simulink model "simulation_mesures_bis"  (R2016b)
settings: Solver=ode15s  StartTime=0.0  StopTime=35*3600  RelTol=1e-3  EnableMultiTasking=on
undefined symbols (not defined in the file or in its folder): C0, C1, Icc, Nbre, Qair, Qpanne, R, R_iso, sigbuilder_block, Time2, V, V0, V1
libraries: powerlib_meascontrol x1, simulink x1

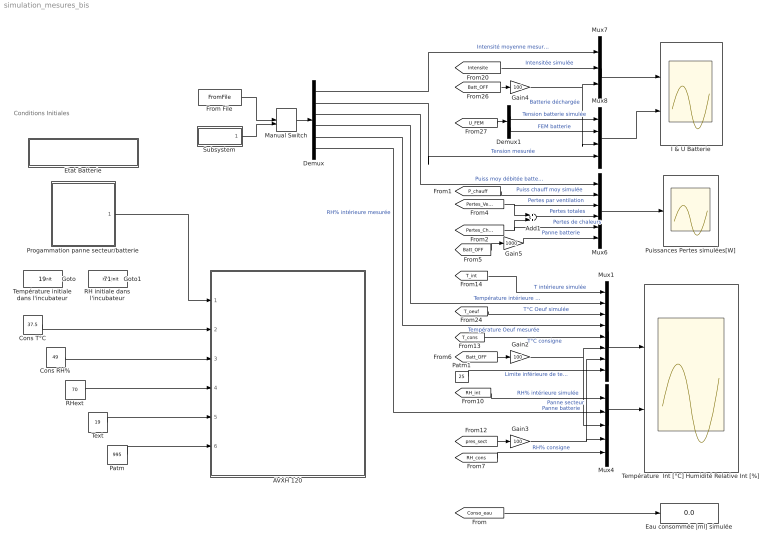
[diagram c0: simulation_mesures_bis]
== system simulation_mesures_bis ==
  note: Conditions Initiales
  AVXH 120 : Subsystem
  Add1 : Sum
  Cons RH% : Constant  Value=49
  Cons T°C : Constant  Value=37.5
  Demux : Demux  Outputs=6
  Demux1 : Demux  Outputs=2
  Eau consommée |ml] simulée : Display
  Etat Batterie : Subsystem  DialogController=hmiCreateDDGDialog  IsWebBlock=on
  From File : FromFile  FileName=mesures1.mat  SampleTime=1
  Gain2 : Gain  Gain=100
  Gain3 : Gain  Gain=100
  Gain4 : Gain  Gain=100
  Gain5 : Gain  Gain=1000
  I & U Batterie : Scope  NumInputPorts=2
  Manual Switch : ManualSwitch
  Mux1 : Mux  Inputs=8
  Mux4 : Mux  Inputs=5
  Mux6 : Mux  Inputs=6
  Mux7 : Mux  Inputs=3
  Mux8 : Mux
  Patm : Constant  Value=995
  Patm1 : Constant  Value=25
  Progammation panne secteur/batterie : Subsystem
  Puissances Pertes simulées[W] : Scope
  RH initiale dans l'incubateur : Constant  Value=71
  RHext : Constant  Value=70
  Subsystem : Subsystem
  Température  Int [°C] Humidité Relative Int [%] : Scope  NumInputPorts=2
  Température initiale dans l'incubateur : Constant  Value=19
  Text : Constant  Value=19
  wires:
  Patm1/1 -> Mux1/8  "Limite inférieure de température"
  Cons T°C/1 -> AVXH 120/2(In2)
  Cons RH%/1 -> AVXH 120/3(In3)
  RHext/1 -> AVXH 120/4(In4)
  Text/1 -> AVXH 120/5(In5)
  Patm/1 -> AVXH 120/6(In6)
  [Conso_eau] -> Eau consommée |ml] simulée/1
  Progammation panne secteur/batterie/1(Out1) -> AVXH 120/1(In1)
  Manual Switch/1 -> Demux/1
  Demux/4 -> Mux1/2  "Température intérieure mesurée"
  Demux/5 -> Mux1/4  "Température Oeuf mesurée"
  Demux/6 -> Mux4/2  "RH% intérieure mesurée"
  [T_int] -> Mux1/1  "T intérieure simulée"
  [Intensite] -> Mux7/2  "Intensitée simulée"
  [RH_int] -> Mux4/1  "RH% intérieure simulée"
  Gain3/1 -> Mux4/4, Mux1/7  "Panne secteur"
  [pres_sect] -> Gain3/1
  [Batt_OFF] -> Gain2/1
  Gain2/1 -> Mux4/3, Mux1/6  "Panne batterie"
  Demux1/1 -> Mux8/1  "Tension batterie simulée"
  [T_cons] -> Mux1/5  "T°C consigne"
  Mux4/1 -> Température  Int [°C] Humidité Relative Int [%]/2
  [P_chauff] -> Mux6/2  "Puiss chauff moy simulée"
  [Pertes_Vent] -> Mux6/3, Add1/1  "Pertes par ventilation"
  Mux6/1 -> Puissances Pertes simulées[W]/1
  [Pertes_Chaleur] -> Mux6/5, Add1/2  "Pertes de chaleurs"
  Add1/1 -> Mux6/4  "Pertes totales"
  [T_oeuf] -> Mux1/3  "T°C Oeuf simulée"
  [RH_cons] -> Mux4/5  "RH% consigne"
  Mux7/1 -> I & U Batterie/1
  Mux8/1 -> I & U Batterie/2
  [U_FEM] -> Demux1/1
  Demux1/2 -> Mux8/2  "FEM batterie"
  [Batt_OFF] -> Gain4/1
  Gain4/1 -> Mux8/3, Mux7/3  "Batterie déchargée"
  [Batt_OFF] -> Gain5/1
  Gain5/1 -> Mux6/6  "Panne batterie"
  Mux1/1 -> Température  Int [°C] Humidité Relative Int [%]/1
  Demux/2 -> Mux8/4  "Tension mesurée"
  Température initiale dans l'incubateur/1 -> [T_init]
  RH initiale dans l'incubateur/1 -> [RH_init]
  Demux/1 -> Mux7/1  "Intensité moyenne mesurée"
  Demux/3 -> Mux6/1  "Puiss moy débitée batterie mesurée"
  From File/1 -> Manual Switch/1
  Subsystem/1(Out1) -> Manual Switch/2

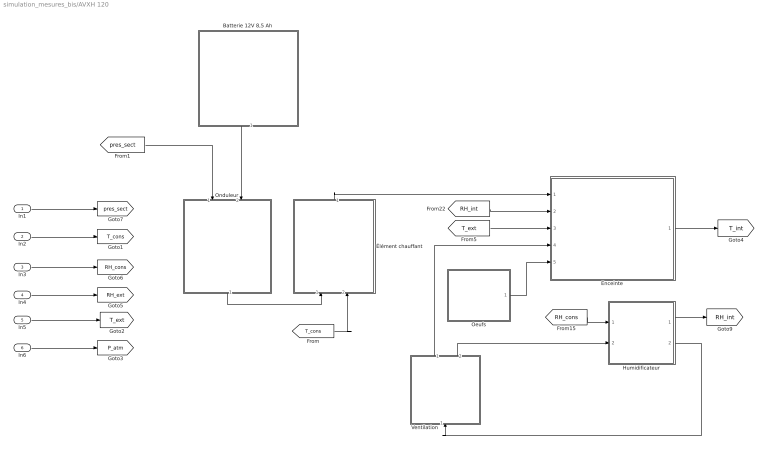
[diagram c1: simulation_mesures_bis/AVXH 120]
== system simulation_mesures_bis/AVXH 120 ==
  In1 : Inport
  In2 : Inport  Port=2
  In3 : Inport  Port=3
  In4 : Inport  Port=4
  In5 : Inport  Port=5
  In6 : Inport  Port=6
  Batterie 12V 8,5 Ah : Subsystem
  Enceinte : Subsystem
  Humidificateur : Subsystem
  Oeufs : Subsystem
  Onduleur : Subsystem
  Ventilation : Subsystem
  Élément chauffant : Subsystem
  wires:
  [RH_int] -> Enceinte/2(In2)
  Enceinte/1(T°C in) -> [T_int]
  In1/1 -> [pres_sect]
  In6/1 -> [P_atm]
  In5/1 -> [T_ext]
  [T_ext] -> Enceinte/3(T°C ext)
  In4/1 -> [RH_ext]
  In3/1 -> [RH_cons]
  Oeufs/1(Out1) -> Enceinte/5(M.Cp_Oeuf)
  [pres_sect] -> Onduleur/1(In1)
  Élément chauffant/1(Out2) -> Enceinte/1(P_chauff)
  Ventilation/1(Out1) -> Enceinte/4(Pertes ventilation)
  [RH_cons] -> Humidificateur/1(In1)
  Ventilation/2(Out2) -> Humidificateur/2(In2)
  Humidificateur/2(Out2) -> Ventilation/1(In1)
  In2/1 -> [T_cons]
  Batterie 12V 8,5 Ah/1(Out3) -> Onduleur/2(In2)
  Onduleur/1(Out1) -> Élément chauffant/1(In1)
  [T_cons] -> Élément chauffant/2(In2)
  Humidificateur/1(Out1) -> [RH_int]

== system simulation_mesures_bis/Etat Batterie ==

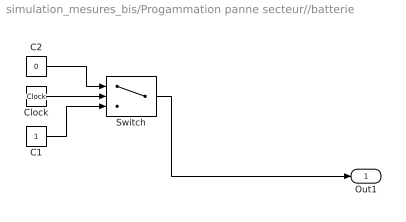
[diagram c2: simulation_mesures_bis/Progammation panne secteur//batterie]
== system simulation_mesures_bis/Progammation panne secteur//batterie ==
  C1 : Constant
  C2 : Constant  Value=0
  Clock : Clock
  Switch : Switch  Criteria=u2 > Threshold  Threshold=Time2
  Out1 : Outport
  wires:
  Clock/1 -> Switch/2
  C2/1 -> Switch/1
  C1/1 -> Switch/3
  Switch/1 -> Out1/1

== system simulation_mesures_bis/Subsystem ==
  Constant : Constant  Value=0
  Mux : Mux  Inputs=6
  Signal Builder : Subsystem  Tag=STV Subsys  LoadFcn=sigbuilder_block('load');  StartFcn=sigbuilder_block('start');  StopFcn=sigbuilder_block('stop');  ClipboardFcn=sigbuilder_block('clipboard');
  Out1 : Outport
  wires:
  Signal Builder/3(RH % int) -> Mux/6
  Signal Builder/1(T°C int) -> Mux/4
  Signal Builder/2(T°C Oeuf) -> Mux/5
  Constant/1 -> Mux/3, Mux/2, Mux/1
  Mux/1 -> Out1/1

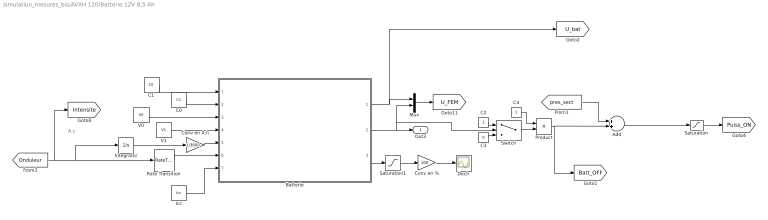
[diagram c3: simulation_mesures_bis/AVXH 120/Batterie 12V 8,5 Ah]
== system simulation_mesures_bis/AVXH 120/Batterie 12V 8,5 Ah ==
  note: A.s
  Add : Sum
  Batterie : MATLAB Function  TreatAsAtomicUnit=on
  C0 : Constant  Value=C1
  C1 : Constant  Value=C0
  C2 : Constant
  C3 : Constant  Value=0
  C4 : Constant
  Conv en % : Gain  Gain=100
  Conv en A.h : Gain  Gain=1/3600
  Dech : Scope
  Icc : Constant  Value=Icc
  Integrator : Integrator
  Mux : Mux  Inputs=2
  Product : Product
  Rate Transition : RateTransition
  Saturation : Saturate  UpperLimit=1  LowerLimit=0
  Saturation1 : Saturate  UpperLimit=1000  LowerLimit=0
  Switch : Switch  Criteria=u2 > Threshold  Threshold=12.0
  V0 : Constant  Value=V0
  V1 : Constant  Value=V1
  Out3 : Outport
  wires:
  Batterie/3(x) -> Saturation1/1
  Conv en %/1 -> Dech/1
  C0/1 -> Batterie/2(C1)
  C1/1 -> Batterie/1(C0)
  V0/1 -> Batterie/3(V0)
  V1/1 -> Batterie/4(V1)
  Icc/1 -> Batterie/7(Icc)
  Integrator/1 -> Conv en A.h/1
  Conv en A.h/1 -> Batterie/5(C)
  Mux/1 -> [U_FEM]
  C2/1 -> Switch/1
  C3/1 -> Switch/3
  Saturation1/1 -> Conv en %/1
  [Onduleur] -> [Intensite], Rate Transition/1, Integrator/1
  Switch/1 -> Product/2
  Saturation/1 -> [Puiss_ON]
  C4/1 -> Product/1
  [pres_sect] -> Add/1
  Batterie/2(E) -> Out3/1, Switch/2, Mux/2
  Add/1 -> Saturation/1
  Product/1 -> Add/2, [Batt_OFF]
  Rate Transition/1 -> Batterie/6(I)
  Batterie/1(U) -> Mux/1, [U_bat]

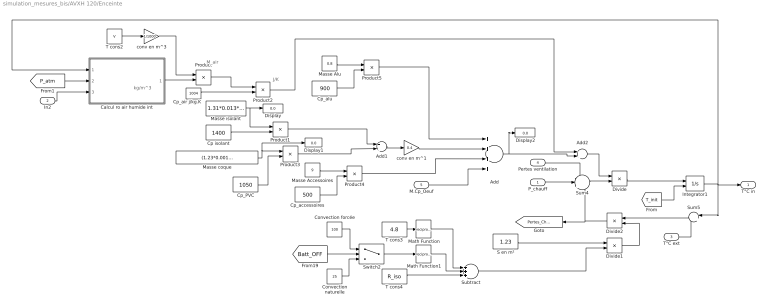
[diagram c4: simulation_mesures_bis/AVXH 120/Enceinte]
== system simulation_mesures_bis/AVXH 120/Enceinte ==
  note: J/K
  note: kg/m^3
  note: M_air
  P_chauff : Inport
  In2 : Inport  Port=2
  T°C ext : Inport  Port=3
  Pertes ventilation : Inport  Port=4
  M.Cp_Oeuf : Inport  Port=5
  Add : Sum  Inputs=++++
  Add1 : Sum
  Add2 : Sum
  Calcul ro air humide int : MATLAB Function  TreatAsAtomicUnit=on
  Convection forcée : Constant  Value=100
  Convection naturelle : Constant  Value=25
  Cp isolant : Constant  Value=1400
  Cp_PVC : Constant  Value=1050
  Cp_accessoires : Constant  Value=500
  Cp_air j/kg.K : Constant  Value=1004
  Cp_alu : Constant  Value=900
  Display : Display
  Display1 : Display
  Display2 : Display
  Divide : Product  Inputs=/*
  Divide1 : Product  Inputs=*/
  Divide2 : Product  Inputs=**
  Integrator1 : Integrator  InitialConditionSource=external  InitialCondition=20
  Masse Accessoires : Constant  Value=9
  Masse Alu : Constant  Value=0.8
  Masse coque : Constant  Value=(1.23*0.001)*1380
  Masse isolant : Constant  Value=1.31*0.013*15
  Math Function : Math  Operator=reciprocal
  Math Function1 : Math  Operator=reciprocal
  Product{,1..5} (6 alike) : Product
  S en m² : Constant  Value=1.23
  Subtract : Sum  Inputs=+++
  Sum4 : Sum  Inputs=-|+|-
  Sum5 : Sum  Inputs=|+-
  Switch2 : Switch  Criteria=u2 > Threshold
  T cons2 : Constant  Value=V
  T cons3 : Constant  Value=4.8
  T cons4 : Constant  Value=R_iso
  conv en m^1 : Gain  Gain=0.4
  conv en m^3 : Gain  Gain=1/1000
  T°C in : Outport
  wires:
  P_chauff/1 -> Sum4/2
  Sum5/1 -> Divide2/1
  Divide2/1 -> Sum4/3, [Pertes_Chaleur]
  T°C ext/1 -> Sum5/2
  T cons2/1 -> conv en m^3/1
  Calcul ro air humide int/1(RO) -> Product/2
  Product/1 -> Product2/1
  Masse isolant/1 -> Display/1, Product1/1
  Cp_air j/kg.K/1 -> Product2/2
  Cp isolant/1 -> Product1/2
  Product1/1 -> Add1/1
  Product2/1 -> Add2/1
  [P_atm] -> Calcul ro air humide int/2(P)
  S en m²/1 -> Divide1/1
  T cons4/1 -> Subtract/3
  Divide1/1 -> Divide2/2
  In2/1 -> Calcul ro air humide int/3(RH)
  Pertes ventilation/1 -> Sum4/1
  conv en m^3/1 -> Product/1
  T cons3/1 -> Math Function/1
  Switch2/1 -> Math Function1/1
  Math Function1/1 -> Subtract/2
  Math Function/1 -> Subtract/1
  Subtract/1 -> Divide1/2
  Cp_PVC/1 -> Product3/2
  Product3/1 -> Add1/2
  Masse Accessoires/1 -> Product4/1
  Cp_accessoires/1 -> Product4/2
  Product4/1 -> Add/3
  Masse Alu/1 -> Product5/1
  Cp_alu/1 -> Product5/2
  Product5/1 -> Add/1
  M.Cp_Oeuf/1 -> Add/4
  [T_init] -> Integrator1/2
  Masse coque/1 -> Display1/1, Product3/1
  Integrator1/1 -> Sum5/1, Calcul ro air humide int/1(T), T°C in/1
  conv en m^1/1 -> Add/2
  Add1/1 -> conv en m^1/1
  Add/1 -> Add2/2, Display2/1
  Divide/1 -> Integrator1/1
  Convection forcée/1 -> Switch2/1
  Convection naturelle/1 -> Switch2/3
  [Batt_OFF] -> Switch2/2
  Sum4/1 -> Divide/2
  Add2/1 -> Divide/1

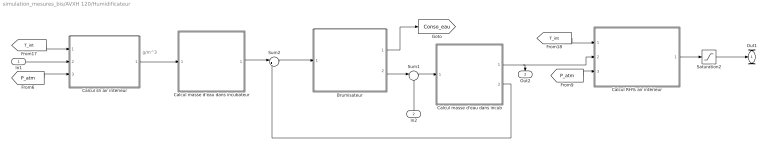
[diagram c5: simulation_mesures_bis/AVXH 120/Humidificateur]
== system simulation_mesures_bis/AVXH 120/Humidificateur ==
  note: g/m^3
  In1 : Inport
  In2 : Inport  Port=2
  Brumisateur : Subsystem
  Calcul RH% air intérieur : MATLAB Function  TreatAsAtomicUnit=on
  Calcul masse d'eau dans incub : Subsystem
  Calcul masse d'eau dans incubateur : Subsystem
  Calcul sh air intérieur : MATLAB Function  TreatAsAtomicUnit=on
  Saturation2 : Saturate  UpperLimit=100  LowerLimit=0
  Sum1 : Sum  Inputs=|++
  Sum2 : Sum  Inputs=|+-
  Out1 : Outport
  Out2 : Outport  Port=2
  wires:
  Sum2/1 -> Brumisateur/1(In1)
  [P_atm] -> Calcul sh air intérieur/3(pl)
  Calcul RH% air intérieur/1(rh) -> Saturation2/1
  Brumisateur/2(Out2) -> Sum1/1
  In1/1 -> Calcul sh air intérieur/2(rh)
  Calcul sh air intérieur/1(sh) -> Calcul masse d'eau dans incubateur/1(In1)
  Calcul masse d'eau dans incub/1(Out1) -> Calcul RH% air intérieur/2(sh), Out2/1
  Sum1/1 -> Calcul masse d'eau dans incub/1(In1)
  [T_int] -> Calcul sh air intérieur/1(T)
  Calcul masse d'eau dans incubateur/1(Out1) -> Sum2/1
  In2/1 -> Sum1/2
  [P_atm] -> Calcul RH% air intérieur/3(pl)
  Brumisateur/1(Out1) -> [Conso_eau]
  Calcul masse d'eau dans incub/2(Out2) -> Sum2/2
  [T_int] -> Calcul RH% air intérieur/1(T)
  Saturation2/1 -> Out1/1

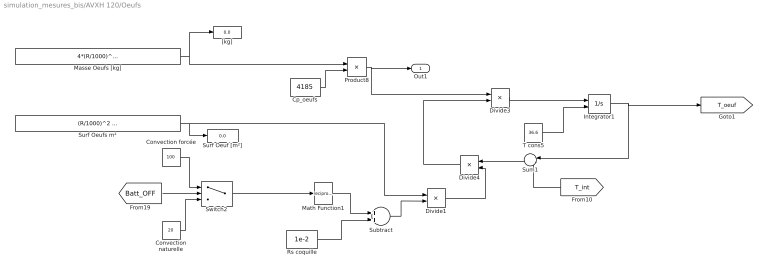
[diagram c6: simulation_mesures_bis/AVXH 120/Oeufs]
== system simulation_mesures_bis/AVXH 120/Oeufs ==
  Convection forcée : Constant  Value=100
  Convection naturelle : Constant  Value=20
  Cp_oeufs : Constant  Value=4185
  Divide1 : Product  Inputs=*/
  Divide3 : Product  Inputs=/*
  Divide4 : Product  Inputs=**
  Integrator1 : Integrator  InitialConditionSource=external  InitialCondition=20
  Masse Oeufs [kg] : Constant  Value=4*(R/1000)^3 * (3.14 * (3 - 1.4142) - 1) *1000*Nbre / 3
  Math Function1 : Math  Operator=reciprocal
  Product8 : Product
  Rs coquille : Constant  Value=1e-2
  Subtract : Sum
  Sum1 : Sum  Inputs=|-+
  Surf Oeuf [m²] : Display
  Surf Oeufs m² : Constant  Value=(R/1000)^2 * (3.14 * (3 - 1.4142) - 1) * Nbre
  Switch2 : Switch  Criteria=u2 > Threshold  Threshold=0.5
  T cons5 : Constant  Value=36.6
  "[kg]" : Display
  Out1 : Outport
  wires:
  Cp_oeufs/1 -> Product8/2
  Product8/1 -> Divide3/1, Out1/1
  Divide4/1 -> Divide3/2
  T cons5/1 -> Integrator1/2
  Integrator1/1 -> [T_oeuf], Sum1/1
  Sum1/1 -> Divide4/1
  Rs coquille/1 -> Subtract/2
  Divide1/1 -> Divide4/2
  Math Function1/1 -> Subtract/1
  Subtract/1 -> Divide1/2
  [T_int] -> Sum1/2
  Divide3/1 -> Integrator1/1
  Surf Oeufs m²/1 -> Divide1/1, Surf Oeuf [m²]/1
  Convection forcée/1 -> Switch2/1
  Convection naturelle/1 -> Switch2/3
  Switch2/1 -> Math Function1/1
  [Batt_OFF] -> Switch2/2
  Masse Oeufs [kg]/1 -> Product8/1, "[kg]"/1

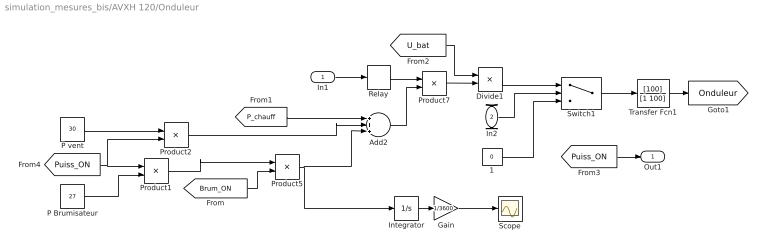
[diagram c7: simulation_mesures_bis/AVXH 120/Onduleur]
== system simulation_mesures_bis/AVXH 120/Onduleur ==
  In1 : Inport
  In2 : Inport  Port=2
  1 : Constant  Value=0
  Add2 : Sum  Inputs=+++
  Divide1 : Product  Inputs=/*
  Gain : Gain  Gain=1/3600
  Integrator : Integrator
  P Brumisateur : Constant  Value=27
  P vent : Constant  Value=30
  Product{1..2,5,7} (4 alike) : Product
  Relay : Relay  OnSwitchValue=1  OffSwitchValue=0  OnOutputValue=0  OffOutputValue=1
  Scope : Scope
  Switch1 : Switch  Threshold=11
  Transfer Fcn1 : TransferFcn  Numerator=[100]  Denominator=[1 100]
  Out1 : Outport
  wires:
  Relay/1 -> Product7/1
  Add2/1 -> Product7/2
  Product2/1 -> Add2/2
  [Brum_ON] -> Product5/2
  Product1/1 -> Product5/1
  Product5/1 -> Integrator/1, Add2/3
  In1/1 -> Relay/1
  [P_chauff] -> Add2/1
  Divide1/1 -> Switch1/1
  1/1 -> Switch1/3
  Product7/1 -> Divide1/2
  [U_bat] -> Divide1/1
  Switch1/1 -> Transfer Fcn1/1
  In2/1 -> Switch1/2
  [Puiss_ON] -> Out1/1
  P Brumisateur/1 -> Product1/2
  [Puiss_ON] -> Product2/2, Product1/1
  P vent/1 -> Product2/1
  Transfer Fcn1/1 -> [Onduleur]
  Integrator/1 -> Gain/1
  Gain/1 -> Scope/1

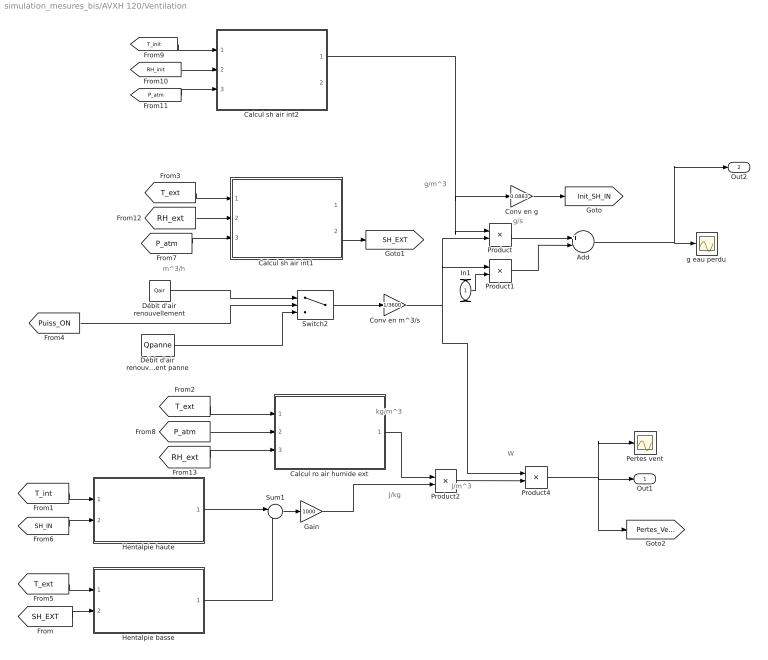
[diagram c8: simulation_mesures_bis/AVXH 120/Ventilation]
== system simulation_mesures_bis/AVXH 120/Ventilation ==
  note: g/s
  note: W
  note: J/m^3
  note: kg/m^3
  note: J/kg
  note: g/m^3
  note: m^3/h
  In1 : Inport
  Add : Sum  Inputs=+-
  Calcul ro air humide ext : MATLAB Function  TreatAsAtomicUnit=on
  Calcul sh air int1 : MATLAB Function  TreatAsAtomicUnit=on
  Calcul sh air int2 : MATLAB Function  TreatAsAtomicUnit=on
  Conv en g : Gain  Gain=0.0883
  Conv en m^3/s : Gain  Gain=1/3600
  Débit d'air renouvellement : Constant  Value=Qair
  Débit d'air renouvellement panne : Constant  Value=Qpanne
  Gain : Gain  Gain=1000
  Hentalpie basse : MATLAB Function  TreatAsAtomicUnit=on
  Hentalpie haute : MATLAB Function  TreatAsAtomicUnit=on
  Pertes vent : Scope
  Product{,1..2,4} (4 alike) : Product
  Sum1 : Sum  Inputs=|+-
  Switch2 : Switch  Criteria=u2 > Threshold
  g eau perdu : Scope
  Out1 : Outport
  Out2 : Outport  Port=2
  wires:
  Add/1 -> Out2/1, g eau perdu/1
  Switch2/1 -> Conv en m^3/s/1
  Conv en m^3/s/1 -> Product1/1, Product/2, Product4/1
  Product/1 -> Add/1
  Product1/1 -> Add/2
  Conv en g/1 -> [Init_SH_IN]
  Calcul ro air humide ext/1(RO) -> Product2/1
  Product2/1 -> Product4/2
  Calcul sh air int2/1(sh) -> Product/1, Conv en g/1
  Débit d'air renouvellement/1 -> Switch2/1
  Débit d'air renouvellement panne/1 -> Switch2/3
  [Puiss_ON] -> Switch2/2
  [T_ext] -> Calcul ro air humide ext/1(T)
  [T_ext] -> Calcul sh air int1/1(T)
  [P_atm] -> Calcul sh air int1/3(pl)
  [P_atm] -> Calcul ro air humide ext/2(P)
  [RH_ext] -> Calcul sh air int1/2(rh)
  [RH_ext] -> Calcul ro air humide ext/3(RH)
  Product4/1 -> [Pertes_Vent], Out1/1, Pertes vent/1
  In1/1 -> Product1/2
  Gain/1 -> Product2/2
  [T_int] -> Hentalpie haute/1(T)
  [T_ext] -> Hentalpie basse/1(T)
  [SH_EXT] -> Hentalpie basse/2(SH)
  [SH_IN] -> Hentalpie haute/2(SH)
  Hentalpie haute/1(H1) -> Sum1/1
  Hentalpie basse/1(H1) -> Sum1/2
  Sum1/1 -> Gain/1
  Calcul sh air int1/2(sh2) -> [SH_EXT]
  [T_init] -> Calcul sh air int2/1(T)
  [RH_init] -> Calcul sh air int2/2(rh)
  [P_atm] -> Calcul sh air int2/3(pl)

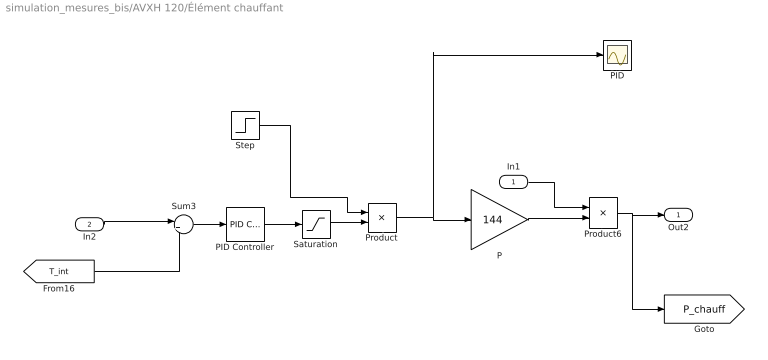
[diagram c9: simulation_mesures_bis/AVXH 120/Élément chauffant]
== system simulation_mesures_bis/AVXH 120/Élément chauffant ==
  In1 : Inport
  In2 : Inport  Port=2
  P : Gain  Gain=144
  PID : Scope
  PID Controller : simulink/Continuous/PID Controller  Controller=PID  TimeDomain=Continuous-time  SampleTime=-1  IntegratorMethod=Forward Euler  FilterMethod=Forward Euler  Form=Parallel  UseFilter=on  ControllerParametersSource=internal  P=0.4  I=0.000031  D=8  N=0.00916449557154445  InitialConditionSource=internal  InitialConditionForIntegrator=0  InitialConditionForFilter=0  ExternalReset=none  LimitOutput=off  UpperSaturationLimit=inf  LowerSaturationLimit=-inf  LinearizeAsGain=on  AntiWindupMode=none  Kb=1  TrackingMode=off  Kt=1  PParamMin=[]  PParamMax=[]  IParamMin=[]  IParamMax=[]  DParamMin=[]  DParamMax=[]  NParamMin=[]  NParamMax=[]  KbParamMin=[]  KbParamMax=[]  KtParamMin=[]  KtParamMax=[]  POutMin=[]  POutMax=[]  IOutMin=[]  IOutMax=[]  DOutMin=[]  DOutMax=[]  NOutMin=[]  NOutMax=[]  KbOutMin=[]  KbOutMax=[]  KtOutMin=[]  KtOutMax=[]  IntegratorOutMin=[]  IntegratorOutMax=[]  FilterOutMin=[]  FilterOutMax=[]  SumOutMin=[]  SumOutMax=[]  SumI1OutMin=[]  SumI1OutMax=[]  SumI2OutMin=[]  SumI2OutMax=[]  SumI3OutMin=[]  SumI3OutMax=[]  SumDOutMin=[]  SumDOutMax=[]  SaturationOutMin=[]  SaturationOutMax=[]  IntegratorContinuousStateAttributes=''  IntegratorStateMustResolveToSignalObject=off  IntegratorRTWStateStorageClass=Auto  FilterContinuousStateAttributes=''  FilterStateMustResolveToSignalObject=off  FilterRTWStateStorageClass=Auto  DifferentiatorICPrevScaledInput=0  DifferentiatorOutMin=[]  DifferentiatorOutMax=[]
  Product : Product
  Product6 : Product
  Saturation : Saturate  UpperLimit=1  LowerLimit=0
  Step : Step  Time=50  SampleTime=0
  Sum3 : Sum  Inputs=|+-
  Out2 : Outport
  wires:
  In2/1 -> Sum3/1
  PID Controller/1 -> Saturation/1
  Sum3/1 -> PID Controller/1
  Saturation/1 -> Product/2
  Product6/1 -> [P_chauff], Out2/1
  [T_int] -> Sum3/2
  In1/1 -> Product6/1
  P/1 -> Product6/2
  Product/1 -> P/1, PID/1
  Step/1 -> Product/1

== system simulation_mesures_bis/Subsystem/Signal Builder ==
  Demux : Demux  Tag=STV Demux  Outputs=3
  FromWs : FromWorkspace  Tag=STV FromWs  VariableName=tuvar  SampleTime=0
  T°C int : Outport  Tag=STV Outport
  T°C Oeuf : Outport  Tag=STV Outport  Port=2
  RH % int : Outport  Tag=STV Outport  Port=3
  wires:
  Demux/1 -> T°C int/1
  FromWs/1 -> Demux/1
  Demux/2 -> T°C Oeuf/1
  Demux/3 -> RH % int/1

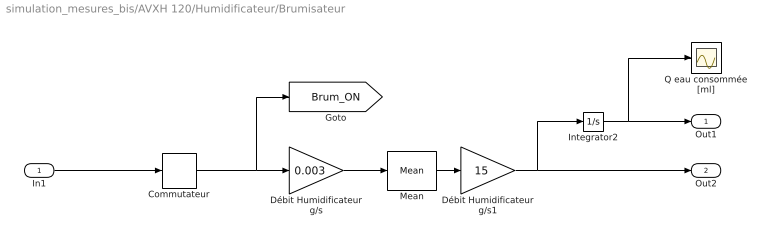
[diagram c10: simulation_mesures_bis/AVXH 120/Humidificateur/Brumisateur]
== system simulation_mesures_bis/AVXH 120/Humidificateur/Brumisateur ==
  In1 : Inport
  Commutateur : Relay  OnSwitchValue=0.12  OffSwitchValue=-0.02
  Débit Humidificateur g/s : Gain  Gain=0.003
  Débit Humidificateur g/s1 : Gain  Gain=15
  Integrator2 : Integrator
  Mean : powerlib_meascontrol/Measurements/Mean  Freq=0.061  Vinit=0  Ts=0
  Q eau consommée [ml] : Scope
  Out1 : Outport
  Out2 : Outport  Port=2
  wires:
  Integrator2/1 -> Q eau consommée [ml]/1, Out1/1
  Commutateur/1 -> Débit Humidificateur g/s/1, [Brum_ON]
  In1/1 -> Commutateur/1
  Débit Humidificateur g/s/1 -> Mean/1
  Mean/1 -> Débit Humidificateur g/s1/1
  Débit Humidificateur g/s1/1 -> Out2/1, Integrator2/1

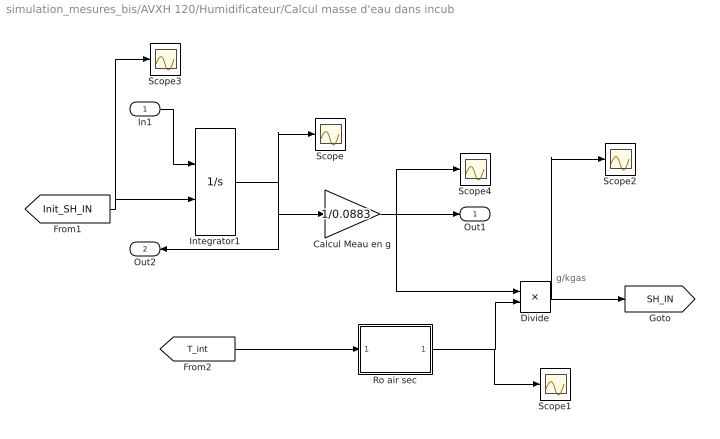
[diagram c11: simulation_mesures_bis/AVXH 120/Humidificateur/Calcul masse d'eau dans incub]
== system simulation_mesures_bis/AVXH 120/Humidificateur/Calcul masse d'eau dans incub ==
  note: g/kgas
  In1 : Inport
  Calcul Meau en g : Gain  Gain=1/0.0883
  Divide : Product  Inputs=*/
  Integrator1 : Integrator  InitialConditionSource=external  InitialCondition=1
  Ro air sec : MATLAB Function  TreatAsAtomicUnit=on
  Scope{,1..4} (5 alike) : Scope
  Out1 : Outport
  Out2 : Outport  Port=2
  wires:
  Calcul Meau en g/1 -> Scope4/1, Divide/1, Out1/1
  In1/1 -> Integrator1/1
  Integrator1/1 -> Calcul Meau en g/1, Out2/1, Scope/1
  [Init_SH_IN] -> Integrator1/2, Scope3/1
  Ro air sec/1(ro) -> Scope1/1, Divide/2
  [T_int] -> Ro air sec/1(T)
  Divide/1 -> Scope2/1, [SH_IN]

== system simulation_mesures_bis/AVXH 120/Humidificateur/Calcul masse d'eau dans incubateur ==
  In1 : Inport
  Calcul Masse eau dans Incub en g : Gain  Gain=0.0883
  Out1 : Outport
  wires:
  In1/1 -> Calcul Masse eau dans Incub en g/1
  Calcul Masse eau dans Incub en g/1 -> Out1/1

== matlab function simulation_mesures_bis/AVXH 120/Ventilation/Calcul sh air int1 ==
function [sh,sh2] =CONV_RH_en_SH(T,rh,pl)

% ######################################################################################################
% function [sh]=goff_gratch(T,rh,pl)
%
% fonction de conversion de l'humidité relative ('rh' : en %)
% en humidité spécifique ('sh' : en g/m^3)
% en fonction de :
% la temperature de l'air ('T' : Kelvin, utiliser la fonction C2K si la T est en °C)
% du niveau pression ('pl' : en hPa, si vous avez des matrices 4D, bouclez sur la dimension 
% niveau). 
%
% utilise l'equation de Goff-Gratch pour la determination de
% la tension de vapeur saturante (es) en fonction de la temperature de l'Air
%
% AUTHOR : Nicolas Fauchereau - CRC Dijon - <nicolasf@u-bourgogne.fr>
%
% ######################################################################################################



%Conversion température
T=T+273;


% tension de vapeur saturante
if (T<0), % par rapport a la glace 
eilog = -9.09718 .* ((273.16 ./ T) -1);
eilog2 = -3.5654 .* log10 (273.16 ./ T);
eilog3 = 0.876793 .* (1 - (T ./ 273.16 ));
es=6.1071 .* 10.^(eilog+eilog2+eilog3);

else, % par rapport à l'eau 
eilog=-7.90298 .* ((373.16 ./ T) - 1);
eilog2=5.02808 .* log10((373.16 ./ T));
eilog3=-1.3816e-7 .* ((10.^(11.344.*(1-(T./373.16)))) -1);
eilog4=8.1328e-3 .* ((10.^( -3.49149 .* ((373.16 ./ T) - 1) )) -1);
es=1013.246 .* 10.^(eilog+eilog2+eilog3+eilog4);
end;


% masse
ws = 0.62197 .* es ./ (pl - 0.378.*es);

% masse volumique
ro = 1.293 .* 273 ./ (T);

% humidité spécifique
sh2 = (rh/100.0) .* ws*1000;
sh=sh2*ro; %%% passage en g.m^3

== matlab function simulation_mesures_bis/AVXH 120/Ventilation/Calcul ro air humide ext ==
function RO = RO_AIR_HUMIDE(T,P,RH)
P=P*100;
RH=RH/100;
RO = 1/(287.06*(T+273.15))*(P-230.617*RH*exp(17.5043*T/(241.2+T)));

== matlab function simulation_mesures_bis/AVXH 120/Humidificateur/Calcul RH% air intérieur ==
function rh  = CONV_SH_en_RH(T,sh,pl)

% ######################################################################################################
% function [sh]=goff_gratch_shtorh(T,sh,pl)
%
% fonction de conversion de l'humidité spécifique ('sh' : en g/m^3)
% en humidité relative ('rh' : %)
% en fonction de :
% la temperature de l'air ('T' : Kelvin, utiliser la fonction C2K si la T est en °C)
% du niveau pression ('pl' : en hPa, si vous avez des matrices 4D, bouclez sur la dimension
% niveau).
%
% utilise l'equation de Goff-Gratch pour la determination de
% la tension de vapeur saturante (es) en fonction de la temperature de l'Air
%
% AUTHOR : Nicolas Fauchereau - CRC Dijon - <nicolasf@u-bourgogne.fr>
%
% ######################################################################################################

%Conversion température
T=T+273;

% tension de vapeur saturante
%if (K2C(T)<0), % par rapport a la glace
if (T<0),
eilog = -9.09718 .* ((273.16 ./ T) -1);
eilog2 = -3.5654 .* log10 (273.16 ./ T);
eilog3 = 0.876793 .* (1 - (T ./ 273.16 ));
es=6.1071 .* 10.^(eilog+eilog2+eilog3);

else, % par rapport à l'eau
eilog=-7.90298 .* ((373.16 ./ T) - 1);
eilog2=5.02808 .* log10((373.16 ./ T));
eilog3=-1.3816e-7 .* ((10.^(11.344.*(1-(T./373.16)))) -1);
eilog4=8.1328e-3 .* ((10.^( -3.49149 .* ((373.16 ./ T) - 1) )) -1);
es=1013.246 .* 10.^(eilog+eilog2+eilog3+eilog4);
end;


% masse
ws = 0.62197 .* es ./ (pl - 0.378.*es);

% masse volumique
ro = 1.293 .* 273 ./ (T);

% humidité relative
rh=(sh./ws) .* 100/(1000*ro);

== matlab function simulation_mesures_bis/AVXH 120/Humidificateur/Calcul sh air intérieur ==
function sh =CONV_RH_en_SH(T,rh,pl)

% ######################################################################################################
% function [sh]=goff_gratch(T,rh,pl)
%
% fonction de conversion de l'humidité relative ('rh' : en %)
% en humidité spécifique ('sh' : en g/m^3)
% en fonction de :
% la temperature de l'air ('T' : Kelvin, utiliser la fonction C2K si la T est en °C)
% du niveau pression ('pl' : en hPa, si vous avez des matrices 4D, bouclez sur la dimension 
% niveau). 
%
% utilise l'equation de Goff-Gratch pour la determination de
% la tension de vapeur saturante (es) en fonction de la temperature de l'Air
%
% AUTHOR : Nicolas Fauchereau - CRC Dijon - <nicolasf@u-bourgogne.fr>
%
% ######################################################################################################



%Conversion température
T=T+273;


% tension de vapeur saturante
if (T<0), % par rapport a la glace 
eilog = -9.09718 .* ((273.16 ./ T) -1);
eilog2 = -3.5654 .* log10 (273.16 ./ T);
eilog3 = 0.876793 .* (1 - (T ./ 273.16 ));
es=6.1071 .* 10.^(eilog+eilog2+eilog3);

else, % par rapport à l'eau 
eilog=-7.90298 .* ((373.16 ./ T) - 1);
eilog2=5.02808 .* log10((373.16 ./ T));
eilog3=-1.3816e-7 .* ((10.^(11.344.*(1-(T./373.16)))) -1);
eilog4=8.1328e-3 .* ((10.^( -3.49149 .* ((373.16 ./ T) - 1) )) -1);
es=1013.246 .* 10.^(eilog+eilog2+eilog3+eilog4);
end;


% masse
ws = 0.62197 .* es ./ (pl - 0.378.*es);

% masse volumique
ro = 1.293 .* 273 ./ (T);

% humidité spécifique
sh = (rh/100.0)*ws;
sh=sh*1000*ro; %%% passage en g.m^3

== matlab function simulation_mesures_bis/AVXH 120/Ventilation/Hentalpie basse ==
function H1 = CALC_HENTALP(T,SH)

H1 =1.006*T+SH*(2500+1.826*T)/1000;

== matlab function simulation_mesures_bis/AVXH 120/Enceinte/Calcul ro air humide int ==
function RO = F(T,P,RH)
P=P*100;
RH=RH/100;
RO = 1/(287.06*(T+273.15))*(P-230.617*RH*exp(17.5043*T/(241.2+T)));

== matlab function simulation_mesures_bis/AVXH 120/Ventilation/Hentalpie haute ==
function H1 = CALC_HENTALP(T,SH)

H1 =1.006*T+SH*(2500+1.826*T)/1000;

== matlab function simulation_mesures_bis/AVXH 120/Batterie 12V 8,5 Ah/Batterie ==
function [U,E,x] = Batterie(C0, C1, V0, V1, C,I, Icc)
%#codegen


x1=C1/C0;
B=(V1-x1*V0)/(V1*(1-x1));
A=1-B;
x=(C0-C)/C0;
V = V0*(1-(A*(1-x))/(1-B*(1-x)));
U=V-V*I/Icc;
E = U/(1-I/Icc);

== matlab function simulation_mesures_bis/AVXH 120/Humidificateur/Calcul masse
d'eau dans incub/Ro air sec ==
function ro = fcn(T)
%#codegen
T=T+273.15;
ro = 1.293 .* 273 ./ (T);

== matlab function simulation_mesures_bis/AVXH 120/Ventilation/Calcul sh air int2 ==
function [sh,sh2] =CONV_RH_en_SH(T,rh,pl)

% ######################################################################################################
% function [sh]=goff_gratch(T,rh,pl)
%
% fonction de conversion de l'humidité relative ('rh' : en %)
% en humidité spécifique ('sh' : en g/m^3)
% en fonction de :
% la temperature de l'air ('T' : Kelvin, utiliser la fonction C2K si la T est en °C)
% du niveau pression ('pl' : en hPa, si vous avez des matrices 4D, bouclez sur la dimension 
% niveau). 
%
% utilise l'equation de Goff-Gratch pour la determination de
% la tension de vapeur saturante (es) en fonction de la temperature de l'Air
%
% AUTHOR : Nicolas Fauchereau - CRC Dijon - <nicolasf@u-bourgogne.fr>
%
% ######################################################################################################



%Conversion température
T=T+273;


% tension de vapeur saturante
if (T<0), % par rapport a la glace 
eilog = -9.09718 .* ((273.16 ./ T) -1);
eilog2 = -3.5654 .* log10 (273.16 ./ T);
eilog3 = 0.876793 .* (1 - (T ./ 273.16 ));
es=6.1071 .* 10.^(eilog+eilog2+eilog3);

else, % par rapport à l'eau 
eilog=-7.90298 .* ((373.16 ./ T) - 1);
eilog2=5.02808 .* log10((373.16 ./ T));
eilog3=-1.3816e-7 .* ((10.^(11.344.*(1-(T./373.16)))) -1);
eilog4=8.1328e-3 .* ((10.^( -3.49149 .* ((373.16 ./ T) - 1) )) -1);
es=1013.246 .* 10.^(eilog+eilog2+eilog3+eilog4);
end;


% masse
ws = 0.62197 .* es ./ (pl - 0.378.*es);

% masse volumique
ro = 1.293 .* 273 ./ (T);

% humidité spécifique
sh2 = (rh/100.0) .* ws*1000;
sh=sh2*ro; %%% passage en g.m^3
